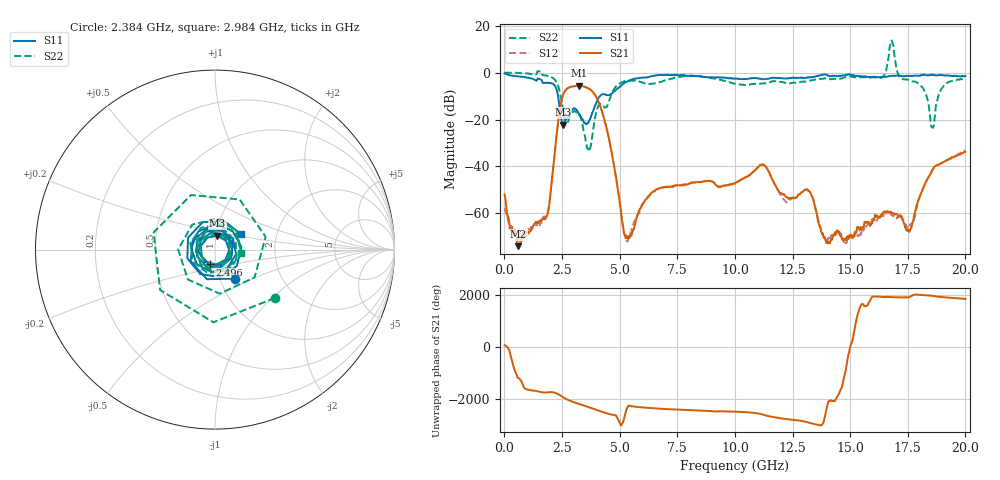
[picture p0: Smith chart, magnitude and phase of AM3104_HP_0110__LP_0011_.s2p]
!Created with skrf (http://scikit-rf.org).
# Hz S RI R 50.0
!freq ReS11 ImS11 ReS21 ImS21 ReS12 ImS12 ReS22 ImS22
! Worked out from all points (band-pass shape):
!   1601 points, 10 MHz to 20 GHz, reference 50 ohm
!   highest |S21| = -5.64 dB at 3.233 GHz (marker M1); lowest = -74.0 dB at 609.7 MHz (marker M2)
!   |S21| within 3 dB of the highest: 2.582 GHz to 3.869 GHz (1.287 GHz wide, 39.9 % of centre)
!   lowest |S11| = -22.1 dB at 2.546 GHz (marker M3), VSWR 1.17, Z = 50.8 + j7.86 ohm
!   |S11| at or under -10 dB: 2.33 GHz to 4.148 GHz (1.818 GHz wide, 56.1 % of centre)
!   |S22| runs from -33.6 to 13.7 dB; largest |S21 - S12| = 0.028
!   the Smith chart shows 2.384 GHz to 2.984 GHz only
!   S11 on the Smith chart (normalised r, x): 2.384 GHz: 1.18, -0.40; 2.496 GHz: 0.93, -0.15; 2.984 GHz: 1.32, +0.23
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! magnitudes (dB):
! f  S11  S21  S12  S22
! 10 MHz  -0.4  -51.9  -57.7  0.0
! 609.7 MHz  -1.6  -74.0  -71.0  -0.1
! 1.847 GHz  -4.4  -61.0  -60.4  -1.3
! 2.384 GHz  -14.1  -17.0  -17.1  -7.3
! 2.496 GHz  -21.1  -11.0  -11.1  -13.0
! 2.546 GHz  -22.1  -9.5  -9.5  -16.0
! 2.984 GHz  -15.5  -5.8  -5.8  -16.6
! 3.233 GHz  -17.5  -5.6  -5.7  -17.9
! 3.346 GHz  -19.4  -5.8  -5.8  -20.0
! 3.683 GHz  -20.3  -6.9  -7.0  -33.6
! 4.27 GHz  -9.2  -17.7  -17.7  -13.9
! 5.295 GHz  -4.0  -69.4  -70.4  -3.4
! 6.682 GHz  -1.1  -49.5  -49.4  -4.3
! 10.01 GHz  -2.7  -47.3  -47.0  -4.8
! 11.2 GHz  -2.8  -39.1  -39.3  -4.6
! 13.34 GHz  -2.0  -52.7  -52.6  -3.3
! 14.04 GHz  -1.3  -72.4  -70.9  -2.7
! 16.68 GHz  -1.6  -59.7  -59.7  7.2
! 17.56 GHz  -1.4  -67.6  -65.6  -3.4
! 18.56 GHz  -0.9  -41.5  -41.7  -23.4
! 19.01 GHz  -1.2  -38.4  -38.2  -6.3
! 20 GHz  -1.5  -33.8  -33.1  -2.5
